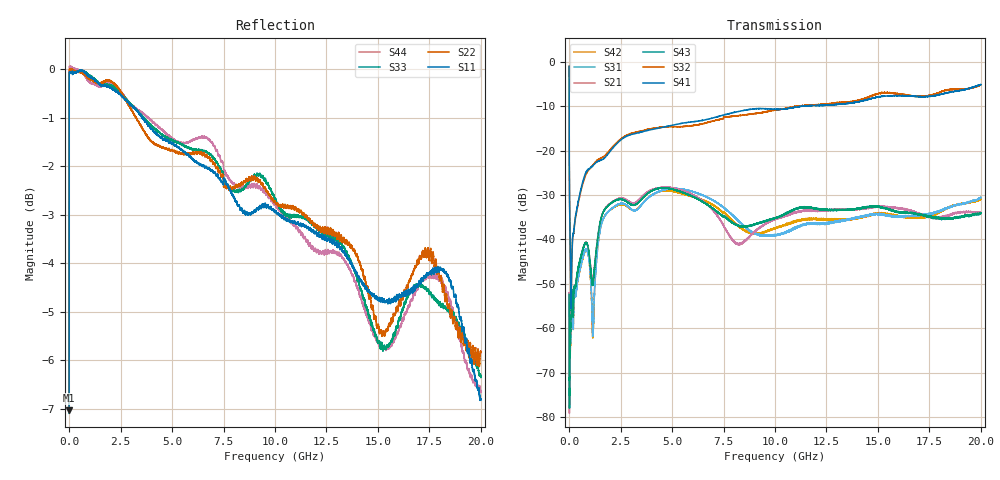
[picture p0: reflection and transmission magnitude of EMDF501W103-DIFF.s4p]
!EMDF501W103
!Johanson Technology Inc.
!www.johansontechnology.com
!Test Board Conditions:
!Substrate Type  RO4350B
!Substrate Thickness  21 mil
!Substrate Dk  3.66
!TL Type: GCPW
!TL Trace Width  40 mil
!TL Gap  17.5 mil
!PART MODE DIFFERENTIAL
!DUT TOPOLOGY	DIFFERENTIAL 4-PORT
# MHz S  dB  R 50
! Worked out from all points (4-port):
!   20001 points, 300 kHz to 20 GHz, reference 50 ohm
!   strongest paths, dB at 300 kHz, 5 GHz, 10 GHz, 15 GHz, 20 GHz:
!     S41: -1.0, -14.3, -10.7, -8.0, -5.1
!     S32: -1.0, -14.6, -10.9, -7.2, -5.2
!     S43: -52.4, -28.7, -35.3, -32.6, -34.1
!     S21: -52.0, -28.4, -35.5, -32.8, -34.1
!     S31: -52.1, -28.6, -39.1, -34.4, -30.6
!     S42: -52.1, -29.1, -37.5, -34.3, -31.0
!   lowest |S11| = -7.0 dB at 300 kHz (marker M1), VSWR 2.60, Z = 25 - j24.6 ohm
!   |S11| at or under -10 dB: nowhere
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0.3  -7.04 -117.3  -52.52 36.3  -53.07 34.1  -1.00 -26.1
     -52.00 36.7  -7.01 -116.9  -1.01 -26.4  -51.65 37.7
     -52.14 37.0  -0.99 -26.1  -7.10 -117.1  -52.09 36.1
     -1.02 -26.2  -52.05 32.1  -52.42 38.8  -6.92 -116.8
142.298  -0.07 178.1  -52.84 71.3  -54.13 67.5  -42.79 67.8
         -52.87 72.5  0.00 178.0  -43.27 67.2  -54.20 69.8
         -54.37 69.3  -43.28 67.3  -0.04 178.2  -52.94 72.0
         -42.83 67.8  -54.44 68.8  -53.03 72.6  0.04 177.8
869.287  -0.10 167.2  -40.95 39.1  -42.36 29.4  -24.55 60.4
         -40.86 39.7  -0.17 167.1  -24.89 63.9  -42.42 28.7
         -42.27 29.7  -24.92 63.7  -0.08 167.2  -41.03 37.6
         -24.52 60.6  -42.65 29.7  -40.97 37.9  -0.20 166.6
1161.283  -0.19 163.2  -48.73 75.8  -61.31 70.4  -23.39 53.0
          -48.93 74.9  -0.24 163.1  -23.22 56.5  -60.94 69.6
          -61.05 68.9  -23.24 56.8  -0.18 163.1  -49.70 75.9
          -23.36 52.9  -60.28 77.0  -49.51 73.9  -0.31 163.3
4203.237  -1.30 122.1  -28.55 -7.7  -29.54 -13.9  -15.03 5.0
          -28.56 -7.7  -1.56 121.8  -14.94 1.6  -29.53 -17.7
          -29.54 -13.8  -14.95 1.6  -1.25 122.9  -28.69 -5.3
          -15.05 5.2  -29.58 -17.5  -28.68 -5.2  -1.16 122.0
11908.12  -3.36 22.5  -33.52 -103.2  -36.58 -153.8  -9.88 -101.5
          -33.57 -103.4  -3.19 24.0  -9.74 -95.1  -35.41 -156.4
          -36.39 -154.1  -9.73 -94.5  -3.24 19.2  -33.03 -111.0
          -9.85 -102.1  -35.39 -156.2  -33.04 -112.2  -3.74 18.6
20000  -6.80 -101.0  -34.49 84.6  -30.67 49.4  -5.34 147.5
       -34.05 84.1  -5.84 -96.6  -4.95 150.8  -31.02 49.2
       -30.56 49.1  -5.17 151.2  -6.34 -98.6  -34.19 84.3
       -5.13 147.0  -30.96 48.9  -34.12 82.9  -6.67 -94.0
